TYPE ST_Status_OutputChn_UINT_TO_BIT :
STRUCT
	Status_of_digital_output		:	BIT;
	Status_of_tristate				:	BIT;
	{attribute 'hide'}
	reserve_b3						:	BIT;
	{attribute 'hide'}
	reserve_b4						:	BIT;
	{attribute 'hide'}
	reserve_b5						:	BIT;
	{attribute 'hide'}
	reserve_b6						:	BIT;
	{attribute 'hide'}
	reserve_b7						:	BIT;
	{attribute 'hide'}
	reserve_b8						:	BIT;
	{attribute 'hide'}
	reserve_byte					:	BYTE;
END_STRUCT
END_TYPE
